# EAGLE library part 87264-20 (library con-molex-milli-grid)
RECEPTACAL
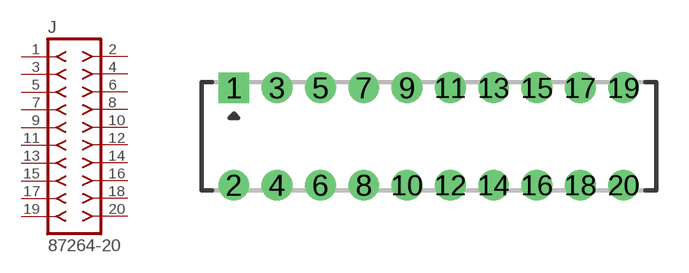
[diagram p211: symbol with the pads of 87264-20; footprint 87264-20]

Designator prefix J

## 87264-20  [87264-20]
1  1  pas
2  2  pas
3  3  pas
4  4  pas
5  5  pas
6  6  pas
7  7  pas
8  8  pas
9  9  pas
10  10  pas
11  11  pas
12  12  pas
13  13  pas
14  14  pas
15  15  pas
16  16  pas
17  17  pas
18  18  pas
19  19  pas
20  20  pas

## Footprint 87264-20 (pad centres in mm)
RECEPTACAL Dual Row, Side Entry
drill 0.914 square: 1 -9,2.25
drill 0.914: 2 -9,-2.25; 3 -7,2.25; 4 -7,-2.25; 5 -5,2.25; 6 -5,-2.25; 7 -3,2.25; 8 -3,-2.25; 9 -1,2.25; 10 -1,-2.25; 11 1,2.25; 12 1,-2.25; 13 3,2.25; 14 3,-2.25; 15 5,2.25; 16 5,-2.25; 17 7,2.25; 18 7,-2.25; 19 9,2.25; 20 9,-2.25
